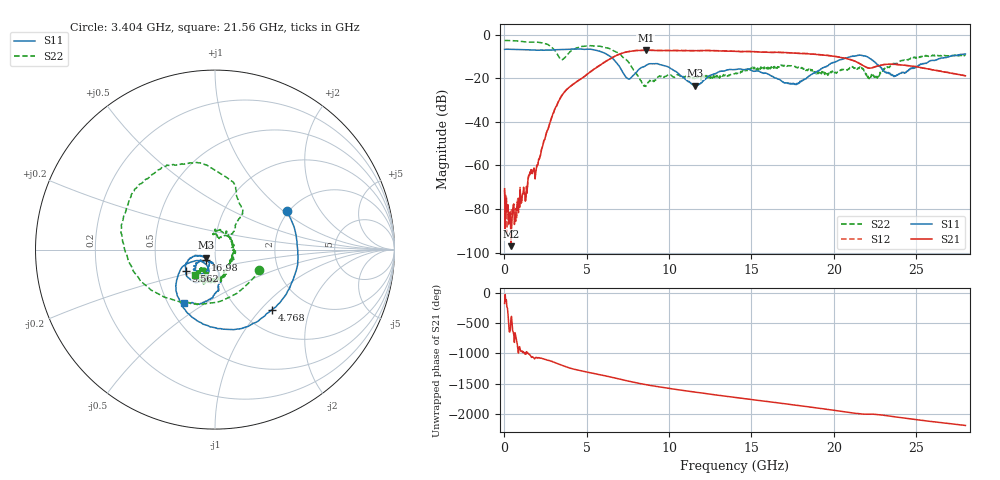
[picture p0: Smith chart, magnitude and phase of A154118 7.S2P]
!  2-Port S-parameters saved by WinCal
! VAR MeasName=S-Parameters (CALIBRATED_DATA) read from VNA (N5230A)
! VAR MeasDate=2015-9-10 14:34:56
! VAR NAME=A154118 7
! VAR FILENAME=A154118 7.S2P
! VAR DATE=2015-9-10 14:34:56
! VAR PHYS_PORTS=1,2
# Hz S DB R 50
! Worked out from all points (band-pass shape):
!   801 points, 10 MHz to 28 GHz, reference 50 ohm
!   highest |S21| = -7.17 dB at 8.582 GHz (marker M1); lowest = -97.0 dB at 394.9 MHz (marker M2)
!   |S21| within 3 dB of the highest: 6.643 GHz to 20.21 GHz (13.56 GHz wide, 101 % of centre)
!   lowest |S11| = -23.4 dB at 11.59 GHz (marker M3), VSWR 1.14, Z = 45 - j4.01 ohm
!   |S11| at or under -10 dB: 6.426 GHz to 21.04 GHz (14.61 GHz wide, 106 % of centre); 21.99 GHz to 27.06 GHz (5.065 GHz wide, 20.7 % of centre)
!   |S22| runs from -23.8 to -2.7 dB; largest |S21 - S12| = 0.0078
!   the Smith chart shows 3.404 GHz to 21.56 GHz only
!   S11 on the Smith chart (normalised r, x): 3.404 GHz: 1.96, +1.05; 4.768 GHz: 1.36, -1.16; 9.562 GHz: 0.70, -0.17; 16.98 GHz: 0.89, -0.11; 21.56 GHz: 0.60, -0.40
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1e7  -6.74 179.5  -70.68 -171.3  -71.31 157.3  -2.66 179.8
3.948625e8  -6.73 163.9  -97.02 -62.4  -86.00 105.8  -2.73 170.3
1.26955e9  -6.96 129.4  -76.32 94.2  -76.34 87.9  -3.33 149.2
2.5291e9  -7.11 73.5  -45.57 -22.9  -45.52 -22.7  -4.18 100.5
3.0889e9  -6.96 45.1  -33.70 -74.3  -33.68 -74.2  -7.53 42.9
3.403788e9  -6.88 28.1  -28.92 -106.0  -28.94 -106.1  -11.34 -24.2
3.823638e9  -6.77 5.4  -24.88 -150.1  -24.84 -149.8  -9.22 -121.9
4.698325e9  -6.64 -43.1  -20.04 147.3  -20.01 147.5  -5.42 166.4
4.7683e9  -6.73 -46.5  -19.71 143.7  -19.66 144.0  -5.39 163.9
6.1678e9  -8.81 -119.8  -12.22 65.2  -12.15 65.0  -6.04 104.7
7.497325e9  -20.22 -133.6  -7.84 -17.4  -7.80 -17.7  -12.14 52.7
8.581938e9  -14.18 -114.8  -7.17 -77.9  -7.13 -78.2  -23.77 73.8
9.351662e9  -13.44 -139.1  -7.32 -113.6  -7.23 -113.9  -19.24 90.7
9.561588e9  -13.95 -144.4  -7.31 -122.3  -7.23 -122.7  -19.22 90.7
1.159086e10  -23.42 -138.8  -7.35 157.8  -7.31 157.2  -19.35 15.4
1.4005e10  -16.06 -125.0  -7.66 70.0  -7.65 69.3  -17.94 -61.4
1.697894e10  -22.01 -131.3  -8.19 -33.4  -8.22 -33.6  -14.38 -111.3
1.869332e10  -18.03 -81.2  -8.91 -94.5  -8.91 -95.0  -16.11 -122.6
2.15623e10  -9.31 -120.6  -13.26 158.4  -13.17 157.0  -15.02 -127.9
2.254195e10  -13.03 -151.6  -14.68 149.2  -14.65 148.2  -19.95 -82.3
2.334666e10  -17.84 -136.4  -13.55 122.3  -13.53 121.1  -14.92 -79.7
2.8e10  -8.89 -109.8  -18.87 -35.3  -18.88 -36.0  -9.16 -120.1
